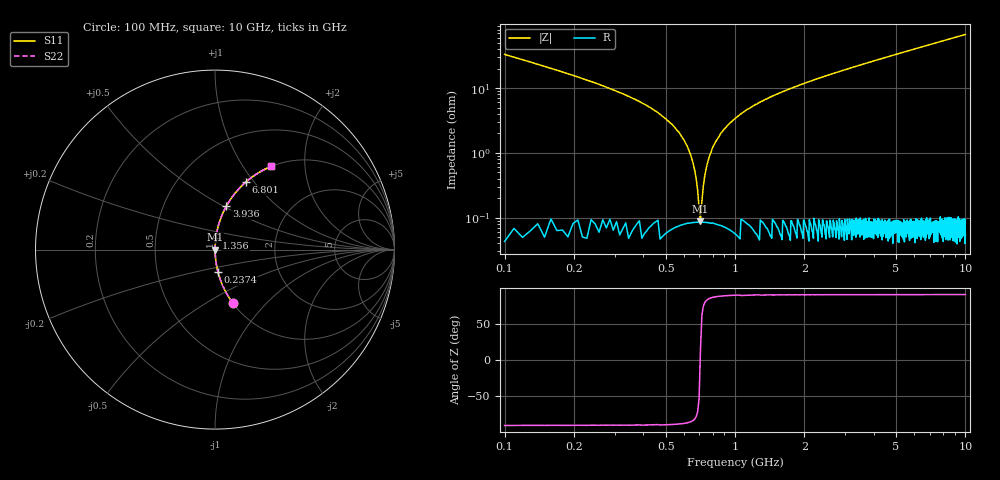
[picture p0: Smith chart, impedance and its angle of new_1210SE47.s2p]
!	AVX	Thin	Film	Operation	Date:	April 2007
!	Description:	Accu-P®	"Series,"	Thin	"Film,"	"SMD,"	RF	Capacitor
!	Part	Number:	12101J470FBT
!	100	MHz	-	5.05	GHz
!	Serial	Measurements
#	MHZ	S	MA	R	50
!	S11	S21	S12	S22
!	dB	Phase	dB	Phase	dB	Phase	dB	Phase
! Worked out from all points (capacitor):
!   1010 points, 100 MHz to 10 GHz, reference 50 ohm
!   read as one part in series: C = 47 pF near 149.1 MHz
!   lowest |Z| = 88 mohm at 708.3 MHz (marker M1)
!   series resonance near 706.7 MHz, so ESL is about 1.1 nH
!   S11 on the Smith chart (normalised r, x): 100 MHz: 1.00, -0.66; 237.4 MHz: 1.00, -0.25; 1.356 GHz: 1.00, +0.13; 3.936 GHz: 1.00, +0.52; 6.801 GHz: 1.00, +0.91; 10 GHz: 1.00, +1.35
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100  0.315 -71.5  0.949 18.3  0.949 18.3  0.315 -71.5
237.364  0.125 -82.5  0.991 7.2  0.991 7.2  0.125 -82.5
443.409  0.046 -86.5  0.998 2.6  0.998 2.6  0.046 -86.5
551.338  0.024 -87.0  0.999 1.4  0.999 1.4  0.024 -87.0
620.02  0.013 -86.1  0.999 0.7  0.999 0.7  0.013 -86.1
678.89  0.00391 -79.5  0.999 0.2  0.999 0.2  0.00391 -79.5
708.325  0.000735 17.8  0.999 -0.0  0.999 -0.0  0.000735 17.8
737.76  0.00418 80.1  0.999 -0.2  0.999 -0.2  0.00418 80.1
777.007  0.00913 85.1  0.999 -0.5  0.999 -0.5  0.00913 85.1
806.442  0.013 86.1  0.999 -0.7  0.999 -0.7  0.013 86.1
904.559  0.024 87.0  0.999 -1.4  0.999 -1.4  0.024 87.0
1090.981  0.043 86.6  0.998 -2.5  0.998 -2.5  0.043 86.6
1355.897  0.067 85.6  0.997 -3.8  0.997 -3.8  0.067 85.6
1758.176  0.099 83.9  0.994 -5.7  0.994 -5.7  0.099 83.9
2444.995  0.15 81.1  0.988 -8.6  0.988 -8.6  0.15 81.1
3406.541  0.216 77.4  0.976 -12.5  0.976 -12.5  0.216 77.4
3936.373  0.25 75.4  0.968 -14.5  0.968 -14.5  0.25 75.4
5054.906  0.318 71.3  0.947 -18.6  0.947 -18.6  0.318 71.3
6703.271  0.41 65.7  0.912 -24.2  0.912 -24.2  0.41 65.7
6801.388  0.415 65.4  0.909 -24.5  0.909 -24.5  0.415 65.4
8351.635  0.49 60.6  0.871 -29.3  0.871 -29.3  0.49 60.6
10000  0.559 56.0  0.829 -34.0  0.829 -34.0  0.559 56.0
